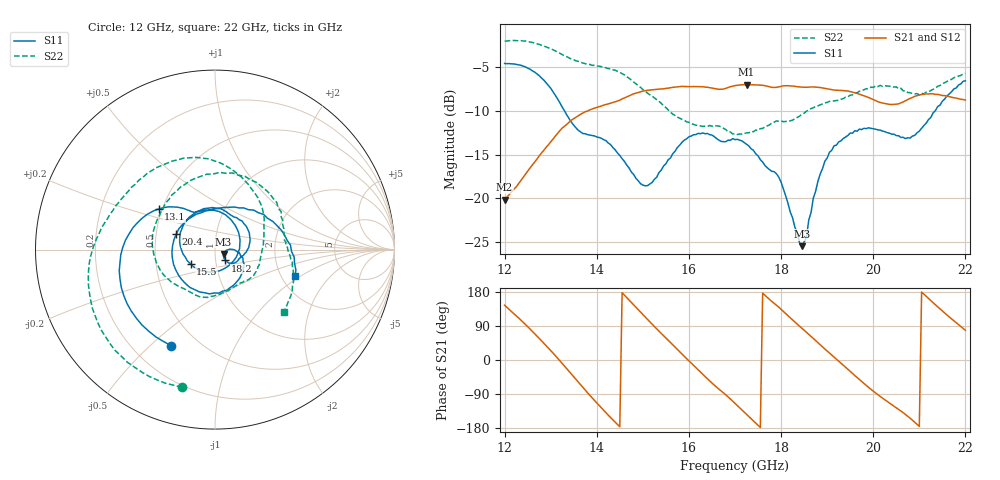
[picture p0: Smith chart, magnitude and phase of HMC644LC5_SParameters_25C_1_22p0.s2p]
!Analog Devices Inc..
!GaAs MMIC 5-BIT DIGITAL PHASE SHIFTER, 15 -8.5 GHz
!Filename: HMC644LC5_sparm_25C_1_0.s2p
!  :25C = 25degC
!  :_1_ = Sn1
!  :_22p0  = 22.5deg
!Device type:
!2 Port Calibration to sma connectors
!Phase Shifter:  0.000
!	TA = +25deg C, 50 Ohm System, Control Voltage = 0/-3V
!Freq	S11	S11	S21	S21	S12	S12	S22	S22
! GHz	Mag dB	Degrees	Mag dB	Degrees	Mag dB	Degrees	Mag dB	Degrees
# GHZ S DB R 50.0
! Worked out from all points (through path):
!   201 points, 12 GHz to 22 GHz, reference 50 ohm
!   highest |S21| = -7.02 dB at 17.25 GHz (marker M1); lowest = -20.1 dB at 12 GHz (marker M2)
!   lowest |S11| = -25.4 dB at 18.45 GHz (marker M3), VSWR 1.11, Z = 54.9 - j2.68 ohm
!   |S11| at or under -10 dB: 13.3 GHz to 21.35 GHz (8.047 GHz wide, 46.5 % of centre)
!   |S22| runs from -12.7 to -2.0 dB; largest |S21 - S12| = 0.0042
!   S11 on the Smith chart (normalised r, x): 12 GHz: 0.36, -0.58; 13.1 GHz: 0.48, +0.25; 15.5 GHz: 0.75, -0.12; 18.2 GHz: 1.11, -0.14; 20.4 GHz: 0.64, +0.12; 22 GHz: 2.37, -0.89
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12  -4.61 -114.5  -20.14 144.5  -20.16 144.6  -2.05 -103.4
12.55  -5.25 -167.6  -16.54 81.9  -16.54 82.0  -2.16 -141.4
13.1  -8.23 144.3  -12.89 11.7  -12.89 11.8  -3.17 -176.8
13.7  -12.60 118.0  -10.25 -72.6  -10.25 -72.6  -4.56 151.0
14.1  -13.14 93.2  -9.46 -126.4  -9.46 -126.2  -4.97 128.8
14.6  -15.78 36.2  -8.54 171.2  -8.54 171.4  -5.90 93.9
15.35  -17.05 -122.3  -7.53 76.1  -7.54 76.3  -8.93 43.8
15.5  -16.05 -149.8  -7.45 58.1  -7.47 58.4  -9.64 34.0
16.15  -12.72 121.8  -7.24 -20.1  -7.23 -19.9  -11.64 -1.3
16.55  -12.95 77.9  -7.46 -66.3  -7.45 -66.2  -11.67 -25.8
17  -13.29 41.8  -7.13 -114.5  -7.13 -114.3  -12.62 -54.6
17.25  -13.82 16.4  -7.02 -143.5  -7.00 -143.6  -12.52 -66.5
17.65  -16.25 -13.9  -7.14 170.7  -7.13 170.8  -11.84 -89.6
18.2  -21.56 -46.5  -7.17 111.2  -7.15 111.1  -11.15 -127.0
18.45  -25.45 -27.1  -7.31 84.1  -7.30 84.0  -10.39 -142.5
18.7  -19.96 0.3  -7.28 57.0  -7.29 56.9  -9.66 -162.9
19.4  -13.00 -62.6  -7.71 -18.9  -7.70 -18.9  -8.45 136.7
19.85  -12.04 -116.3  -8.39 -67.2  -8.38 -67.2  -7.49 96.3
20.35  -12.56 166.8  -9.27 -113.7  -9.25 -113.5  -7.20 49.1
20.4  -12.67 158.2  -9.29 -117.8  -9.29 -117.6  -7.21 45.9
21.15  -11.41 59.7  -8.08 168.1  -8.07 168.1  -7.87 1.6
22  -6.58 -18.2  -8.78 78.4  -8.84 78.2  -5.72 -42.1
